// 伺服轴控制功能块
FUNCTION_BLOCK FB_Axis_PTP
VAR_INPUT
	AXIS			:	REFERENCE TO ST_AXIS_DATA;
END_VAR
VAR
	fbPower			:	MC_Power;
	fbJog			:	MC_Jog;
	fbReset			:	MC_Reset;
	fbMoveAbs		:	MC_MoveAbsolute;
	fbMoveVelo		:	MC_MoveVelocity;
	fbSetPos		:	MC_SetPosition;
	fbGearIn		:	MC_GearIn;
	fbGearOut		:	MC_GearOut;
	fbStop			:	MC_Stop;
	fbHome			:	MC_Home;
END_VAR



Axis.AXIS_REF.ReadStatus();
fbPower(
	Axis:= AXIS.AXIS_REF, 
	Enable:= AXIS.bEnable, 
	Enable_Positive:= TRUE, 
	Enable_Negative:= TRUE, 
	Override:= 100, 
	BufferMode:= , 
	Options:= , 
	Status=> AXIS.bEnabled, 
	Busy=> , 
	Active=> , 
	Error=> , 
	ErrorID=> );
fbJog(
	Axis:= AXIS.AXIS_REF, 
	JogForward:= AXIS.bJogForward, 
	JogBackwards:= AXIS.bJogBackward, 
	Mode:= AXIS.eMode, 
	Position:= AXIS.rPosition, 
	Velocity:= AXIS.rVelocity, 
	Acceleration:= , 
	Deceleration:= , 
	Jerk:= , 
	Done=> , 
	Busy=> , 
	Active=> , 
	CommandAborted=> , 
	Error=> , 
	ErrorID=> );
fbReset(
	Axis:= AXIS.AXIS_REF, 
	Execute:= AXIS.bResetAxis, 
	Done=> , 
	Busy=> , 
	Error=> , 
	ErrorID=> );
fbMoveAbs(
	Axis:= AXIS.AXIS_REF, 
	Execute:= AXIS.bMoveAbs, 
	Position:= AXIS.rPosition, 
	Velocity:= AXIS.rVelocity, 
	Acceleration:= , 
	Deceleration:= , 
	Jerk:= , 
	BufferMode:= , 
	Options:= , 
	Done=> , 
	Busy=> , 
	Active=> , 
	CommandAborted=> , 
	Error=> , 
	ErrorID=> );
fbMoveVelo(
	Axis:= AXIS.AXIS_REF, 
	Execute:= AXIS.bMoveVelo, 
	Velocity:= AXIS.rVelocity, 
	Acceleration:= , 
	Deceleration:= , 
	Jerk:= , 
	Direction:= , 
	BufferMode:= , 
	Options:= , 
	InVelocity=> , 
	Busy=> , 
	Active=> , 
	CommandAborted=> , 
	Error=> , 
	ErrorID=> );
fbSetPos(
	Axis:= AXIS.AXIS_REF, 
	Execute:= , 
	Position:= , 
	Mode:= , 
	Options:= , 
	Done=> , 
	Busy=> , 
	Error=> , 
	ErrorID=> );
IF __ISVALIDREF(AXIS.refMaster) THEN 
	fbGearIn(
		Master:= AXIS.refMaster, 
		Slave:= AXIS.AXIS_REF, 
		Execute:= AXIS.bGearIn, 
		RatioNumerator:= AXIS.RatioNumerator, 
		RatioDenominator:= AXIS.RatioDenominator, 
		Acceleration:= , 
		Deceleration:= , 
		Jerk:= , 
		BufferMode:= , 
		Options:= , 
		InGear=> , 
		Busy=> , 
		Active=> , 
		CommandAborted=> , 
		Error=> , 
		ErrorID=> );
	fbGearOut(
		Slave:= AXIS.AXIS_REF, 
		Execute:= AXIS.bGearOut, 
		Options:= , 
		Done=> , 
		Busy=> , 
		Error=> , 
		ErrorID=> );
END_IF
fbStop(
	Axis:= AXIS.AXIS_REF, 
	Execute:= AXIS.bStop, 
	Deceleration:= , 
	Jerk:= , 
	Options:= , 
	Done=> , 
	Busy=> , 
	Active=> , 
	CommandAborted=> , 
	Error=> , 
	ErrorID=> );
fbHome(
	Axis:= AXIS.AXIS_REF, 
	Execute:= AXIS.bHome, 
	Position:= , 
	HomingMode:= MC_DefaultHoming, 
	BufferMode:= , 
	Options:= , 
	bCalibrationCam:= AXIS.bHomeCam, 
	Done=> , 
	Busy=> , 
	Active=> , 
	CommandAborted=> , 
	Error=> , 
	ErrorID=> );

END_FUNCTION_BLOCK
